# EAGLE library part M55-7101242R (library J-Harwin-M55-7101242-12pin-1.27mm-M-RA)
Harwin M55-7101242R A 12 pin 1.27 mm male SMT connector with plastic alignment pins. Note: alignment pin hole diameters are 0.05 mm smaller than recommended in order to tighten up connector location; this requires hand placement of this package.
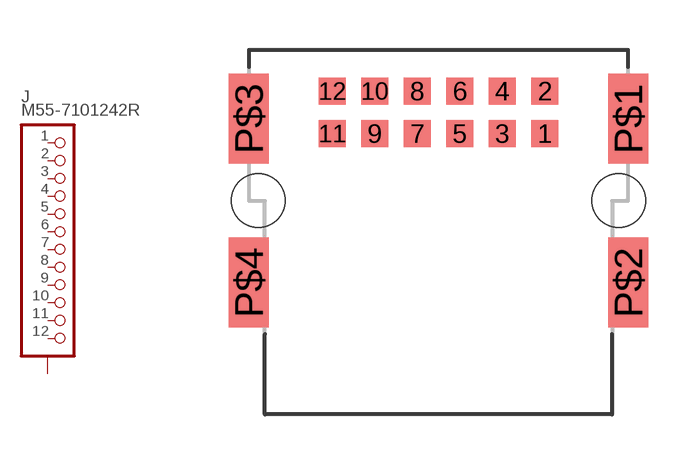
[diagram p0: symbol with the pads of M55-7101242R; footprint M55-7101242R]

Designator prefix J

## M55-7101242R  [M55-7101242R]
1  1  pas
2  2  pas
3  3  pas
4  4  pas
5  5  pas
6  6  pas
7  7  pas
8  8  pas
9  9  pas
10  10  pas
11  11  pas
12  12  pas
P$1  SHIELD  pas
P$2  SHIELD  pas
P$3  SHIELD  pas
P$4  SHIELD  pas

## Footprint M55-7101242R (pad centres in mm)
Harwin M55-7101242R A 12 pin 1.27 mm male SMT connector with plastic alignment pins. Note: alignment pin hole diameters are 0.05 mm smaller than recommended in order to tighten up connector location;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
smd 0.8 x 0.8: 1 3.175,2; 2 3.175,3.27; 3 1.905,2; 4 1.905,3.27; 5 0.635,2; 6 0.635,3.27; 7 -0.635,2; 8 -0.635,3.27; 9 -1.905,2; 10 -1.905,3.27; 11 -3.175,2; 12 -3.175,3.27
smd 1.2 x 2.7: P$1 5.67,2.45; P$2 5.67,-2.45; P$3 -5.67,2.45; P$4 -5.67,-2.45
hole 1.6 at 5.385,0
hole 1.6 at -5.385,0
